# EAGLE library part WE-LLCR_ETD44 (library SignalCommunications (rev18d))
WE-LLCR Resonant Converter Characteristics Transformer for high efficiency power supply Input voltage 360–400 VDC Switching frequency 70–120 kHz Output power 150 W–250 W Testing voltage 4 kVAC Litz wire for low eddy current losses Defined leakage inductance for use without additional resonant inductor Applications Power supplies for PC, netbook, LED lighting and other power supplies High efficient resonant converters Details see: http://katalog.we-online.de/en/pbs/WE-LLCR? Updated by Dan Xu 2014-07-07 2014 (C) Wurth Elektronik
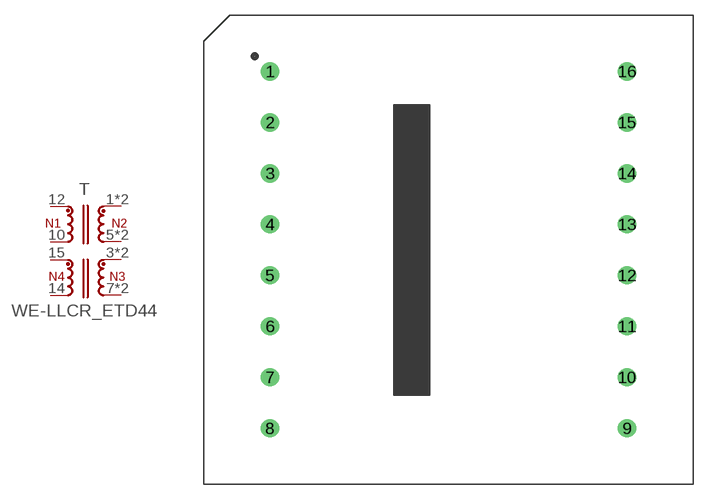
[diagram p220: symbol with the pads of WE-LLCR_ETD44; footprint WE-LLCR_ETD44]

Designator prefix T

## WE-LLCR_ETD44_760895731, WE-LLCR_ETD44_760895741, WE-LLCR_ETD44_760895751  [WE-LLCR_ETD44]
1  2  pas
2  2  pas
3  4  pas
4  4  pas
5  3  pas
6  3  pas
7  5  pas
8  5  pas
10  8  pas
12  1  pas
14  6  pas
15  7  pas

## Footprint WE-LLCR_ETD44 (pad centres in mm)
size: ETD39 Height : 27.5mm max
drill 1.2: 1 -17.5,17.5; 2 -17.5,12.5; 3 -17.5,7.5; 4 -17.5,2.5; 5 -17.5,-2.5; 6 -17.5,-7.5; 7 -17.5,-12.5; 8 -17.5,-17.5; 9 17.5,-17.5; 10 17.5,-12.5; 11 17.5,-7.5; 12 17.5,-2.5; 13 17.5,2.5; 14 17.5,7.5; 15 17.5,12.5; 16 17.5,17.5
